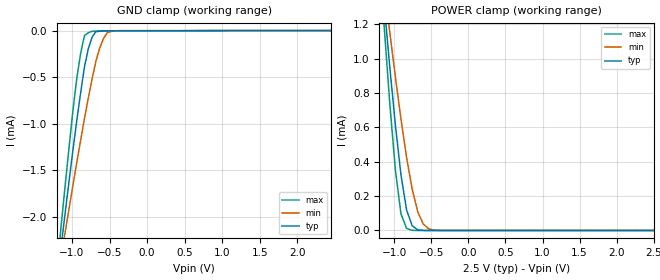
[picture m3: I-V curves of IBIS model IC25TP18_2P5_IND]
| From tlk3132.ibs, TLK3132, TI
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|   Model Cell IC25TP18_2P5_IND
|IC25TP18_2P5
[Model]   IC25TP18_2P5_IND
Model_type   Input
Polarity   Non-Inverting
Vinl =  0.7V
Vinh =  1.7V
C_comp   0.5354074p   0.4896019p   0.590865p
[Model Spec]
Vinl   0.7V   0.7V   0.7V
Vinh   1.7V   1.7V   1.7V
[Temperature Range]   25   125   -40
[Voltage Range]   2.5   2.375   2.625
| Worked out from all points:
|   GND clamp passes 1 mA (typ) near -0.94 V on its own axis
|   POWER clamp passes 1 mA (typ) near -1.07 V on its own axis
[POWER_clamp]
|   voltage   I(typ)   I(min)   I(max)
-2.5V     8.347mA    6.555mA    9.999mA
-1.136V   1.318mA    1.424mA    1.191mA
-1.111V   1.197mA    1.335mA    1.042mA
-1.061V   954.2uA    1.155mA    742.5uA
-984.8mV  614.8uA    894.5uA    353.8uA
-909.1mV  323.2uA    648.1uA    96.22uA
-833.3mV  118.7uA    424.7uA    12.28uA
-757.6mV  27.16uA    238.5uA    711.9nA
-681.8mV  3.612uA    106.7uA    59.28nA
-606.1mV  316.7nA    35.89uA    39.53nA
-530.3mV  42.27nA    8.572uA    38.19nA
2.5V      20.19nA    31.68nA    32.61nA
[GND_clamp]
|   voltage   I(typ)   I(min)   I(max)
-2.5V     -11.64mA   -9.341mA   -13.38mA
-1.187V   -2.612mA   -2.648mA   -2.458mA
-1.136V   -2.269mA   -2.396mA   -2.039mA
-1.086V   -1.932mA   -2.146mA   -1.631mA
-934.3mV  -960.6uA   -1.413mA   -506.4uA
-833.3mV  -389.9uA   -945.2uA   -53.67uA
-782.8mV  -197.5uA   -727.3uA   -24.19uA
-732.3mV  -71.7uA    -522.4uA   -8.043uA
-631.3mV  -6.205uA   -189.2uA   -5.05uA
-530.3mV  -2.384uA   -22.59uA   -4.926uA
-479.8mV  -2.348uA   -9.655uA   -4.906uA
2.449V    19.91nA    32.33nA    30.88nA
